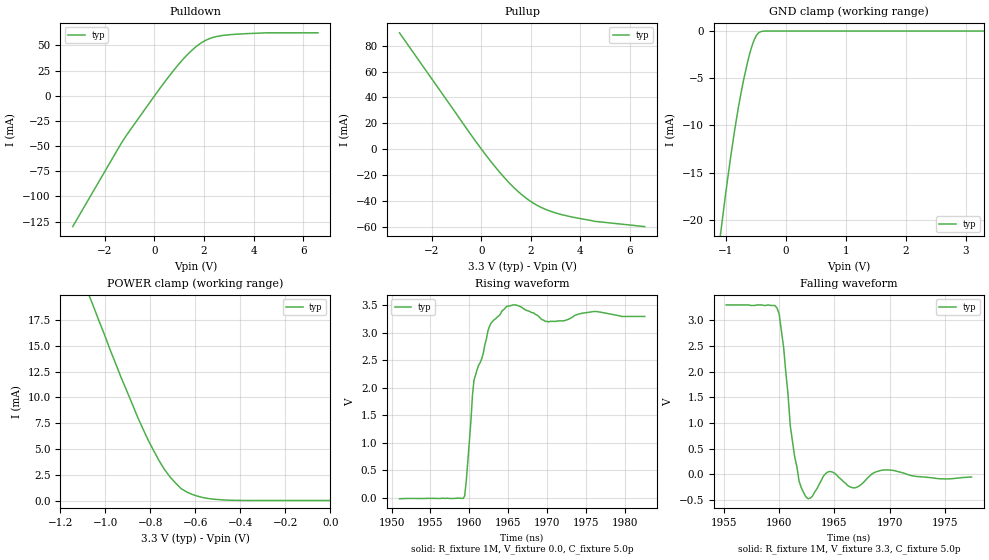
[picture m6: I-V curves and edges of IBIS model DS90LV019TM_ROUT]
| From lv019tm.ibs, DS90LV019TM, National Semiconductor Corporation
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|   Receiver Output MODEL {START}
[Model]   DS90LV019TM_ROUT
Model_type   3-state
|Signals   ROUT
Vmeas = 1.5V   |Reference voltage for timing measurements
Cref = 5pF   |Timing specification test load capacitance value
Rref = 50   |Note: 100 Ohm between the two driver outputs
Vref = 1.2   |Timing specification test load voltage; GND
|   typ   min   max
C_comp   3.07pF   NA   NA
|   typ   min   max
[Temperature Range]   25.0   NA   NA
[Voltage range]   3.3V   3.0V   3.6V
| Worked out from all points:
|   slope of the pulldown table from 0 to 0.495 V, typ, clamps not added: 30 ohm
|   slope of the pullup table from 0 to 0.495 V, typ, clamps not added: 40.1 ohm
|   GND clamp passes 1 mA (typ) near -0.53 V on its own axis
|   POWER clamp passes 1 mA (typ) near -0.65 V on its own axis
|   rising waveform, R_fixture 1M, V_fixture 0.0, C_fixture 5.0p: 20-80 % time 2.01ns typ, NA min, NA max; typ from -0.021 V to 3.3 V
|   falling waveform, R_fixture 1M, V_fixture 3.3, C_fixture 5.0p: 20-80 % time 915ps typ, NA min, NA max; typ from 3.3 V to -0.05 V
[Pulldown]
| Voltage   I(typ)   I(min)   I(max)
-3.3V     -130mA     NA         NA
-1.378V   -48.82mA   NA         NA
-1.011V   -35.14mA   NA         NA
93mV      2.951mA    NA         NA
705mV     23.03mA    NA         NA
1.194V    37.32mA    NA         NA
1.685V    48.85mA    NA         NA
1.93V     53.14mA    NA         NA
2.175V    56.23mA    NA         NA
2.787V    59.95mA    NA         NA
4.502V    62.46mA    NA         NA
6.6V      62.46mA    NA         NA
[Pullup]
|  Voltage   I(typ)   I(min)   I(max)
| Note that the[Pullup]voltage table is referenced to Vcc
| and is calculated using Vtable=Vcc - Vmeasured.
-3.3V     90mA       NA         NA
-467mV    12.51mA    NA         NA
146mV     -3.542mA   NA         NA
636mV     -15.45mA   NA         NA
1.004V    -23.56mA   NA         NA
1.371V    -30.77mA   NA         NA
1.738V    -36.89mA   NA         NA
2.35V     -44.49mA   NA         NA
2.718V    -47.55mA   NA         NA
3.207V    -50.54mA   NA         NA
4.555V    -55.88mA   NA         NA
6.6V      -60mA      NA         NA
[Power_clamp]
| Note that the[POWER_clamp]voltage table is referenced to Vcc
| and is calculated using Vtable=Vcc - Vmeasured.
| Voltage   I(typ)   I(min)   I(max)
-3.3V     140mA      NA         NA
-1.079V   20.26mA    NA         NA
-1.054V   18.89mA    NA         NA
-932mV    12.04mA    NA         NA
-859mV    8.21mA     NA         NA
-810mV    5.865mA    NA         NA
-736mV    2.969mA    NA         NA
-711mV    2.244mA    NA         NA
-663mV    1.148mA    NA         NA
-589mV    411.5uA    NA         NA
-515mV    117.4uA    NA         NA
0V        1.048uA    NA         NA
[GND_clamp]
|Voltage   I(typ)   I(min)   I(max)
-3.3V     -140mA     NA         NA
-1.103V   -22.15mA   NA         NA
-1.072V   -20.61mA   NA         NA
-980mV    -16.07mA   NA         NA
-858mV    -10.65mA   NA         NA
-797mV    -8.274mA   NA         NA
-705mV    -5.173mA   NA         NA
-613mV    -2.637mA   NA         NA
-552mV    -1.335mA   NA         NA
-491mV    -462.8uA   NA         NA
-429mV    -90.16uA   NA         NA
3.3V      524.2nA    NA         NA
[Ramp]
|   typ   min   max
dV/dt_r   1.97/2.09ns   NA   NA
dV/dt_f   1.97/1.0ns   NA   NA
R_load = 100Ohm
|D019ror
[Rising Waveform]
R_fixture = 1M
V_fixture = 0.0
C_fixture = 5.0p | Jig capacitance
|   Time   V(Typ)   V(Min)   V(Max)
1.951us   -21.2mV    NA         NA
1.959us   27.8mV     NA         NA
1.961us   2.14V      NA         NA
1.962us   2.53V      NA         NA
1.963us   3.12V      NA         NA
1.965us   3.48V      NA         NA
1.967us   3.48V      NA         NA
1.97us    3.2V       NA         NA
1.976us   3.39V      NA         NA
1.983us   3.3V       NA         NA
|d019rof
[Falling Waveform]
R_fixture = 1M
V_fixture = 3.3
C_fixture = 5.0p | Jig capacitance
|   Time   V(Typ)   V(Min)   V(Max)
1.955us   3.3V       NA         NA
1.96us    3.24V      NA         NA
1.96us    2.47V      NA         NA
1.961us   947mV      NA         NA
1.961us   344mV      NA         NA
1.963us   -471mV     NA         NA
1.965us   59.4mV     NA         NA
1.967us   -262mV     NA         NA
1.969us   86.2mV     NA         NA
1.977us   -50mV      NA         NA
